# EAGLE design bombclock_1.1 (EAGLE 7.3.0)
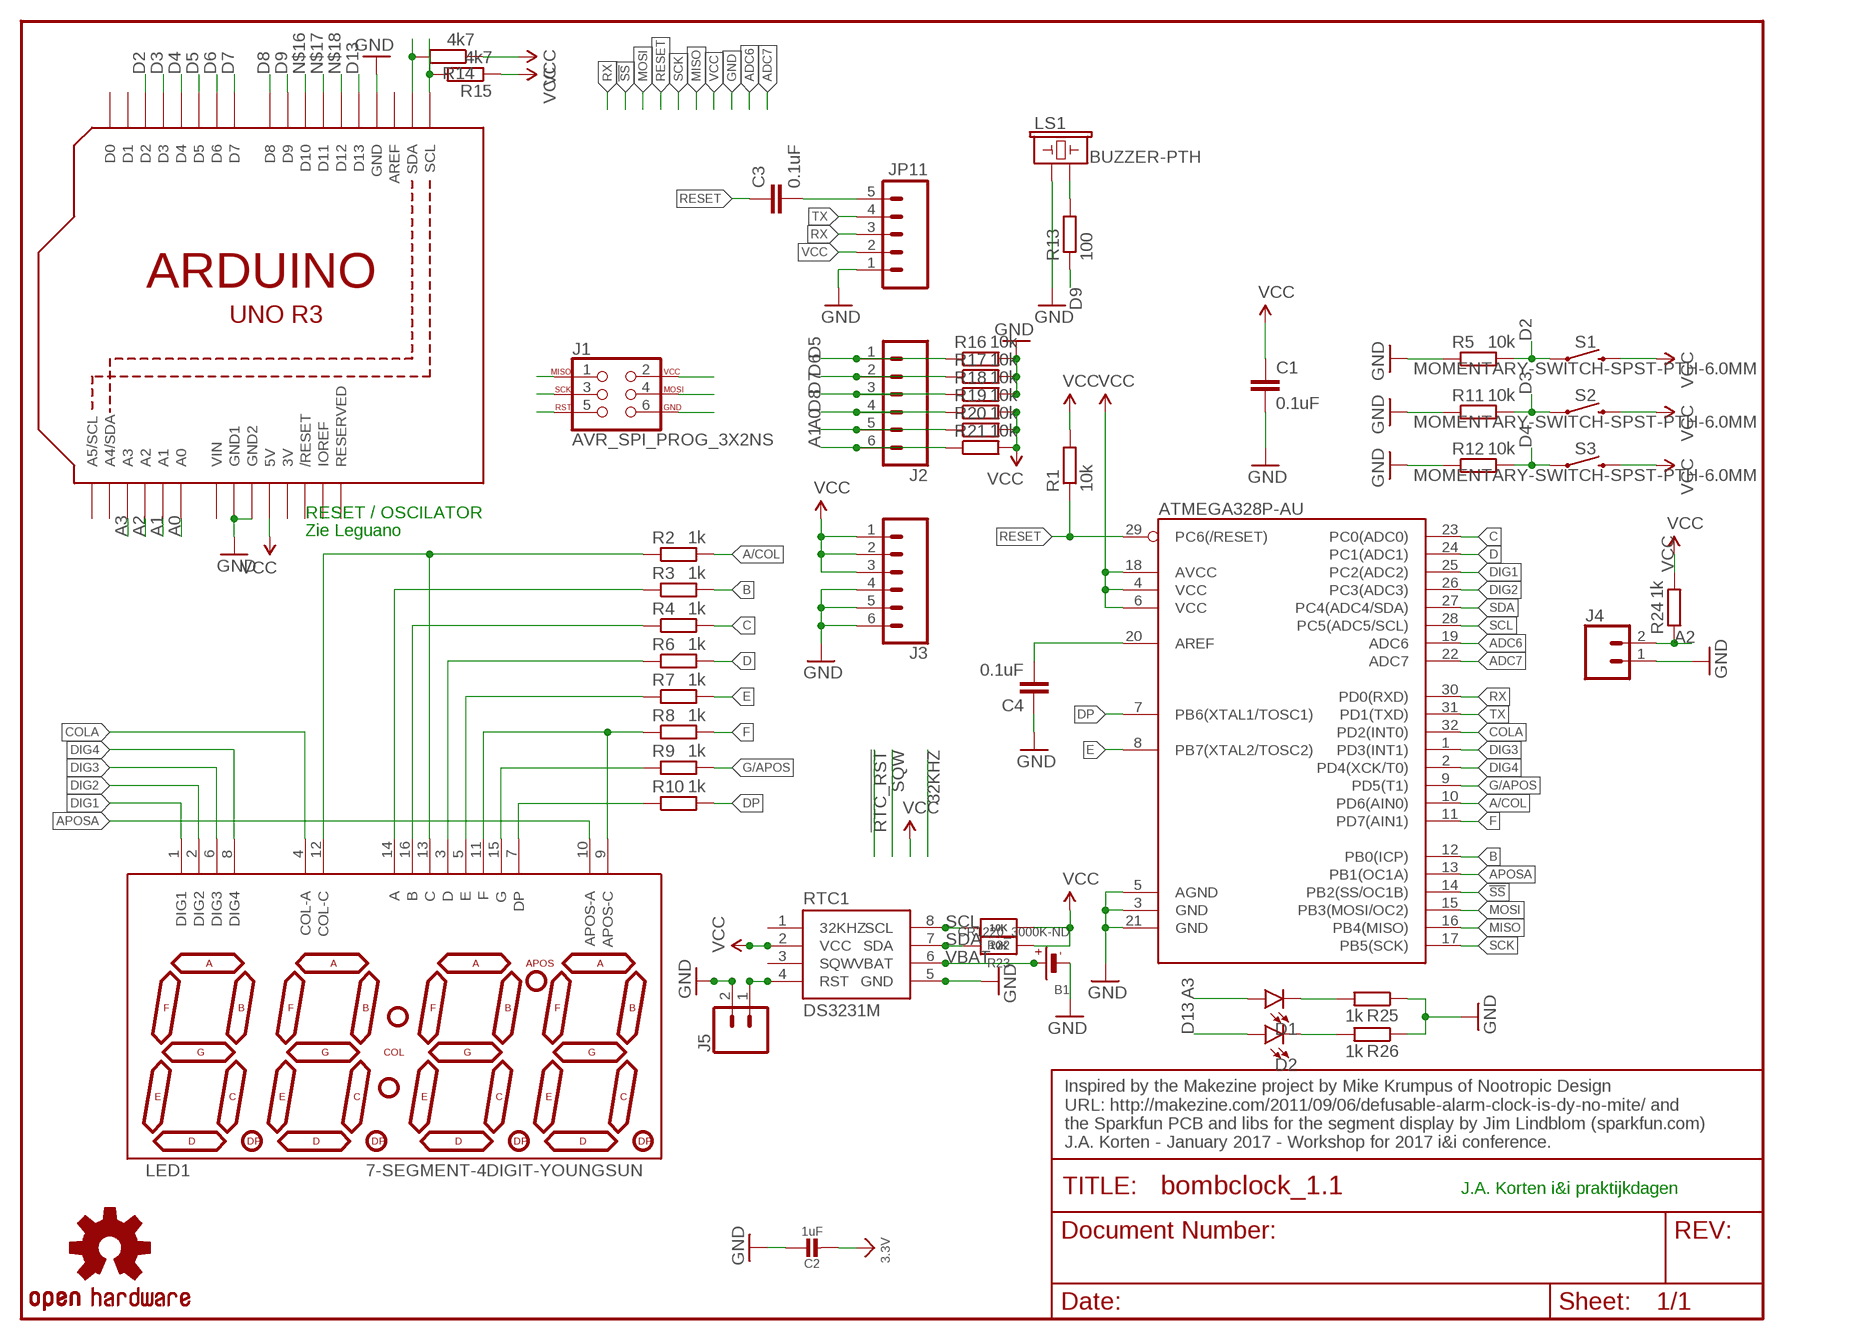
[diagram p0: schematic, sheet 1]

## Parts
ATMEGA328P-AU  ATMEGA328P-AU  ATMEGA168  [TQFP32-08]
B1  CR1220_3000K-ND  BATTERYCR1220_SMT  [CR1220]
C1  0.1uF  CAP0402-CAP  [0402-CAP]
C2  1uF  CAP_CERAMIC0805-NOOUTLINE  [0805-NO]
C3  0.1uF  CAP0402-CAP  [0402-CAP]
C4  0.1uF  CAP0402-CAP  [0402-CAP]
D1  LED5MM  [LED_5MM]
D2  LED5MM  [LED_5MM]
J1  AVR_SPI_PROG_3X2NS  [2X3-NS]
J2  CONN_06SILK_FEMALE_PTH  [1X06]
J3  CONN_06SILK_FEMALE_PTH  [1X06]
J4  CONN_02  [1X02]
J5  CONN_02  [1X02]
JP11  M05PTH-NS  [1X05_NO_SILK]
LED1  7-SEGMENT-4DIGIT-YOUNGSUN  [7-SEGMENT-4DIGIT-YOUNGSUN]
LS1  BUZZER-PTH  [BUZZER-12MM]
R1  10k  R-EU_R0603  [R0603]
R2  1k  R-EU_R0603  [R0603]
R3  1k  R-EU_R0603  [R0603]
R4  1k  R-EU_R0603  [R0603]
R5  10k  R-EU_R0603  [R0603]
R6  1k  R-EU_R0603  [R0603]
R7  1k  R-EU_R0603  [R0603]
R8  1k  R-EU_R0603  [R0603]
R9  1k  R-EU_R0603  [R0603]
R10  1k  R-EU_R0603  [R0603]
R11  10k  R-EU_R0603  [R0603]
R12  10k  R-EU_R0603  [R0603]
R13  100  R-EU_R0603  [R0603]
R14  4k7  R-EU_R0603  [R0603]
R15  4k7  R-EU_R0603  [R0603]
R16  10k  R-EU_R0603  [R0603]
R17  10k  R-EU_R0603  [R0603]
R18  10k  R-EU_R0603  [R0603]
R19  10k  R-EU_R0603  [R0603]
R20  10k  R-EU_R0603  [R0603]
R21  10k  R-EU_R0603  [R0603]
R22  10K  RESISTOR0805_NOOUTLINE  [0805-NO]
R23  10K  RESISTOR0805_NOOUTLINE  [0805-NO]
R24  1k  R-EU_R0603  [R0603]
R25  1k  R-EU_R0603  [R0603]
R26  1k  R-EU_R0603  [R0603]
RTC1  DS3231M  [SO08]
S1  MOMENTARY-SWITCH-SPST-PTH-6.0MM  [TACTILE_SWITCH_PTH_6.0MM]
S2  MOMENTARY-SWITCH-SPST-PTH-6.0MM  [TACTILE_SWITCH_PTH_6.0MM]
S3  MOMENTARY-SWITCH-SPST-PTH-6.0MM  [TACTILE_SWITCH_PTH_6.0MM]
U1  ARDUINOR3-DIMENSION  [ARDUINOR3]
U$4  OSHW-LOGOS  [OSHW-LOGO-S]

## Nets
3.3V: C2.2
!SS: ATMEGA328P-AU.14(PB2(SS/OC1B))
A0: J2.5 R20.1 U1.A0
A1: J2.6 R21.1 U1.A1
A2: J4.2 R24.1 U1.A2
A3: D1.A U1.A3
A/COL: ATMEGA328P-AU.10(PD6(AIN0)) R2.2
ADC6: ATMEGA328P-AU.19(ADC6)
ADC7: ATMEGA328P-AU.22(ADC7)
APOSA: ATMEGA328P-AU.13(PB1(OC1A)) LED1.10(APOS-A)
B: ATMEGA328P-AU.12(PB0(ICP)) R3.2
C: ATMEGA328P-AU.23(PC0(ADC0)) R4.2
COLA: ATMEGA328P-AU.32(PD2(INT0)) LED1.4(COL-A)
D: ATMEGA328P-AU.24(PC1(ADC1)) R6.2
D2: R5.2 S1.1 U1.D2
D3: R11.2 S2.1 U1.D3
D4: R12.2 S3.1 U1.D4
D5: J2.1 R16.1 U1.D5
D6: J2.2 R17.1 U1.D6
D7: J2.3 R18.1 U1.D7
D8: J2.4 R19.1 U1.D8
D9: R13.1 U1.D9
D13: D2.A U1.D13
DIG1: ATMEGA328P-AU.25(PC2(ADC2)) LED1.1(DIG1)
DIG2: ATMEGA328P-AU.26(PC3(ADC3)) LED1.2(DIG2)
DIG3: ATMEGA328P-AU.1(PD3(INT1)) LED1.6(DIG3)
DIG4: ATMEGA328P-AU.2(PD4(XCK/T0)) LED1.8(DIG4)
DP: ATMEGA328P-AU.7(PB6(XTAL1/TOSC1)) R10.2
E: ATMEGA328P-AU.8(PB7(XTAL2/TOSC2)) R7.2
F: ATMEGA328P-AU.11(PD7(AIN1)) R8.2
G/APOS: ATMEGA328P-AU.9(PD5(T1)) R9.2
GND: ATMEGA328P-AU.3(GND) ATMEGA328P-AU.5(AGND) ATMEGA328P-AU.21(GND) B1.- C1.2 C2.1 C4.1 J1.6 J3.4 J3.5 J3.6 J4.1 J5.2 JP11.1 LS1.+ R5.1 R11.1 R12.1 R16.2 R17.2 R18.2 R25.1 R26.1 RTC1.5(GND) U1.GND U1.GND1 U1.GND2
MISO: ATMEGA328P-AU.16(PB4(MISO)) J1.1
MOSI: ATMEGA328P-AU.15(PB3(MOSI/OC2)) J1.4
N$1: ATMEGA328P-AU.20(AREF) C4.2
N$2: LED1.7(DP) R10.1
N$3: LED1.15(G) R9.1
N$4: LED1.9(APOS-C) LED1.11(F) R8.1
N$5: LED1.5(E) R7.1
N$6: LED1.3(D) R6.1
N$8: LED1.16(B) R4.1
N$9: LED1.14(A) R3.1
N$10: LED1.12(COL-C) LED1.13(C) R2.1
N$12: D1.K(C) R25.2
N$13: C3.2 JP11.5
N$14: D2.K(C) R26.2
N$16: U1.D10
N$17: U1.D11
N$18: U1.D12
N$20: LS1.- R13.2
PP: J5.1 RTC1.4(RST)
RESET: ATMEGA328P-AU.29(PC6(/RESET)) C3.1 J1.5 R1.1
RX: ATMEGA328P-AU.30(PD0(RXD)) JP11.3
SCK: ATMEGA328P-AU.17(PB5(SCK)) J1.3
SCL: ATMEGA328P-AU.28(PC5(ADC5/SCL)) R15.2 R22.2 RTC1.8(SCL) U1.SCL
SDA: ATMEGA328P-AU.27(PC4(ADC4/SDA)) R14.2 R23.2 RTC1.7(SDA) U1.SDA
TX: ATMEGA328P-AU.31(PD1(TXD)) JP11.4
VBAT: B1.+$1(+) RTC1.6(VBAT)
VCC: ATMEGA328P-AU.4(VCC) ATMEGA328P-AU.6(VCC) ATMEGA328P-AU.18(AVCC) C1.1 J1.2 J3.1 J3.2 J3.3 JP11.2 R1.2 R14.1 R15.1 R19.2 R20.2 R21.2 R22.1 R23.1 R24.2 RTC1.2(VCC) S1.3 S2.3 S3.3 U1.5V
Unconnected: RTC1.1(32KHZ) RTC1.3(SQW) U1.A4(A4/SDA) U1.A5(A5/SCL) U1.AREF U1.D0 U1.D1 U1.IOREF U1.RESERVED U1.RESET(/RESET)

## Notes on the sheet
- RESET / OSCILATOR
- Zie Leguano
- Inspired by the Makezine project by Mike Krumpus of Nootropic Design 
  URL: http://makezine.com/2011/09/06/defusable-alarm-clock-is-dy-no-mite/ and 
  the Sparkfun PCB and libs for the segment display by Jim Lindblom (sparkfun.com)
  J.A. Korten - January 2017 - Workshop for 2017 i&i conference.
- J.A. Korten i&i praktijkdagen

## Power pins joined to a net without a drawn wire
3V: U1.3V
VIN: U1.VIN

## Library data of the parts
ATMEGA328P-AU = SparkFun:ATMEGA168
B1 = microbuilder:BATTERY: CR1220 SMT - Digikey: 3001K-ND
C1 = SparkFun:CAP: Capacitor
C2 = microbuilder:CAP_CERAMIC: Ceramic Capacitors
C3 C4 = SparkFun-Passives:CAP: Capacitor
D1 D2 = SparkFun-LED:LED: LED (Generic)
J1 = SparkFun-Connectors:AVR_SPI_PROG_3X2: AVR ISP 6 Pin This is the reduced ISP connector for AVR programming. Common on Arduino. This footprint will take up less PCB space and can be used with a 10-pin to 6-pin adapter such as SKU: BOB-08508 **Special note about "TEST_POINT" package. The stop mask is on the top side, so if you want your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
J2 J3 = SparkFun-Connectors:CONN_06: Multi connection point. Often used as Generic Header-pin footprint for 0.1 inch spaced/style header connections On any of the 0.1 inch spaced packages, you can populate with these: Break Away Headers - Straight (PRT-00116) Break Away Male Headers - Right Angle (PRT-00553) Female Headers (PRT-00115)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; PROD_ID: CONN-08437
J4 J5 = SparkFun-Connectors:CONN_02: Multi connection point. Often used as Generic Header-pin footprint for 0.1 inch spaced/style header connections
JP11 = SparkFun-Connectors:M05: Header 5 Standard 5-pin 0.1" header. Use with straight break away headers (SKU : PRT-00116), right angle break away headers (PRT-00553), swiss pins (PRT-00743), machine pins (PRT-00117), and female headers (PRT-00115). Molex polarized connector foot print use with SKU : PRT-08230 with associated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
LED1 = SparkFun:7-SEGMENT-4DIGIT-YOUNGSUN: This is a part for the 4-Digit 7-segment LEDs from Young Sun. Different from the Digikey LEDs, all 16 pins are used. The LONGPADS Variant is used for a test jig, but you may like it because there is more pad to solder to. If you are concerned about routing space, the standard works just fine though.
LS1 = SparkFun-Electromechanical:BUZZER: Buzzer; PROD_ID: COMP-08253; SF_SKU: COM-07950
R1-R21 R24-R26 = rcl:R-EU_: RESISTOR, European symbol
R22 R23 = microbuilder:RESISTOR: Resistors
RTC1 = SparkFun-Clocks:DS3231M: DS3231M Real Time Clock Accuracy +/-5ppm. Battery Backup. 2.3V to 5.5V. Datasheet SparkFun Products CryptoCape (DEV-12773) SparkFun CryptoShield (DEV-13183); PROD_ID: IC-11985
S1-S3 = SparkFun-Switches:MOMENTARY-SWITCH-SPST: Momentary Switch (Pushbutton) - SPST; PROD_ID: SWCH-08441; SF_SKU: COM-00097
U1 = adafruit:ARDUINOR3: This is a new object for the new Arduino R3 - with extra pins that you may want to use (such as IOref, and duplicated A4/A5
U$4 = SparkFun-Aesthetics:OSHW-LOGO: Open Source Hardware Logo This logo indicates the piece of hardware it is found on incorporates a OSHW license and/or adheres to the definition of open source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

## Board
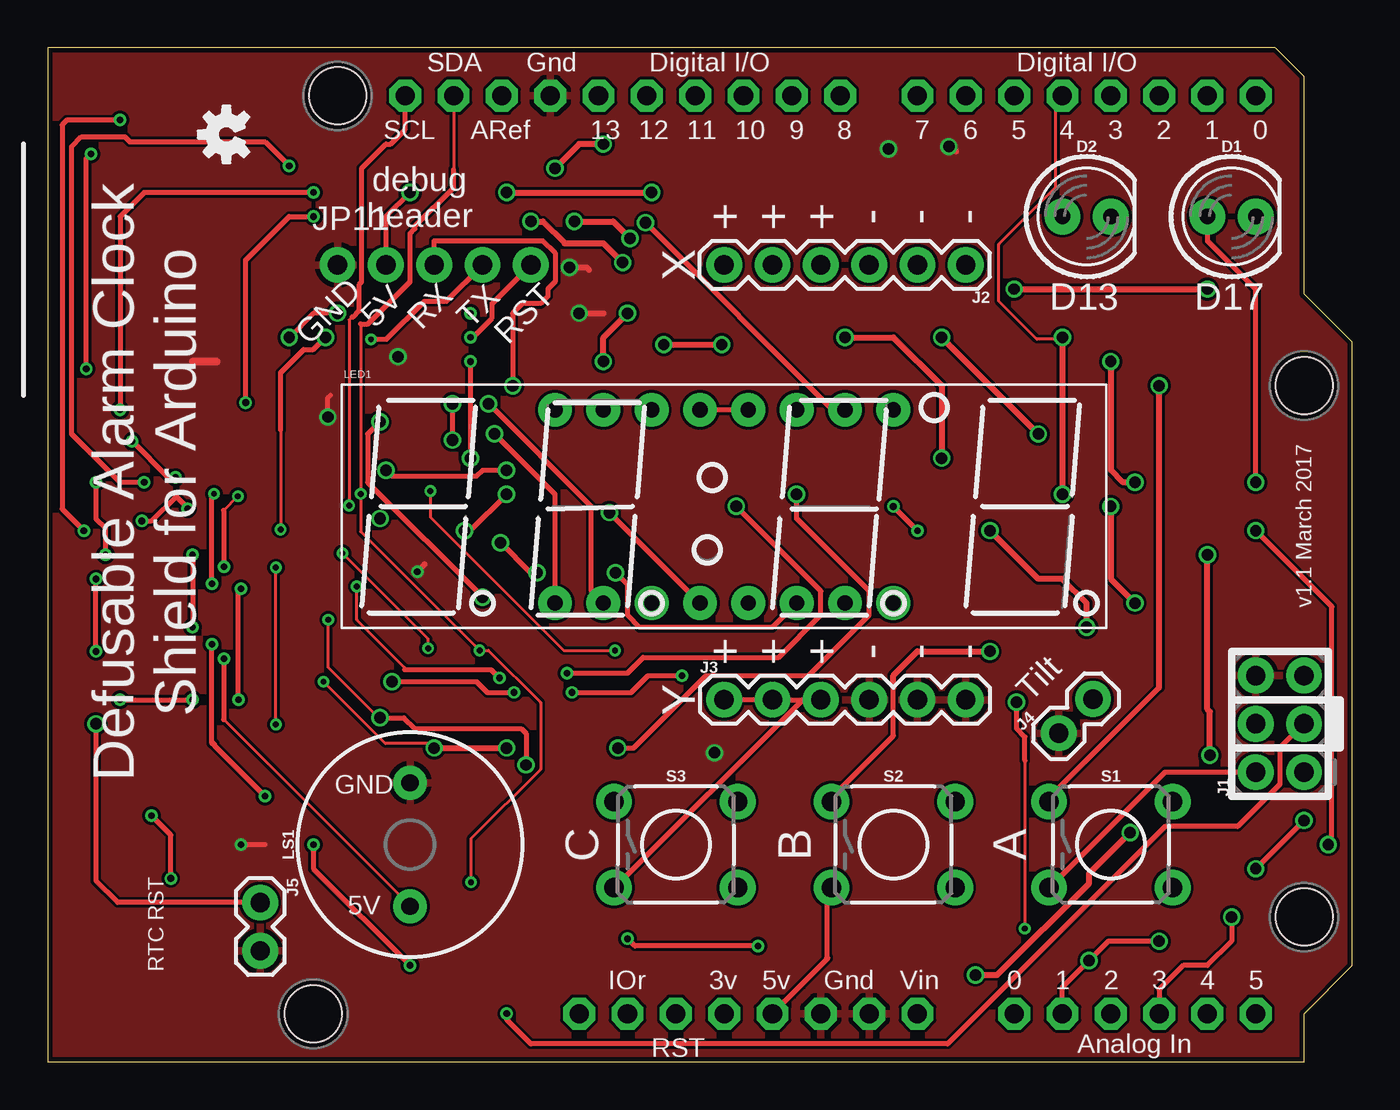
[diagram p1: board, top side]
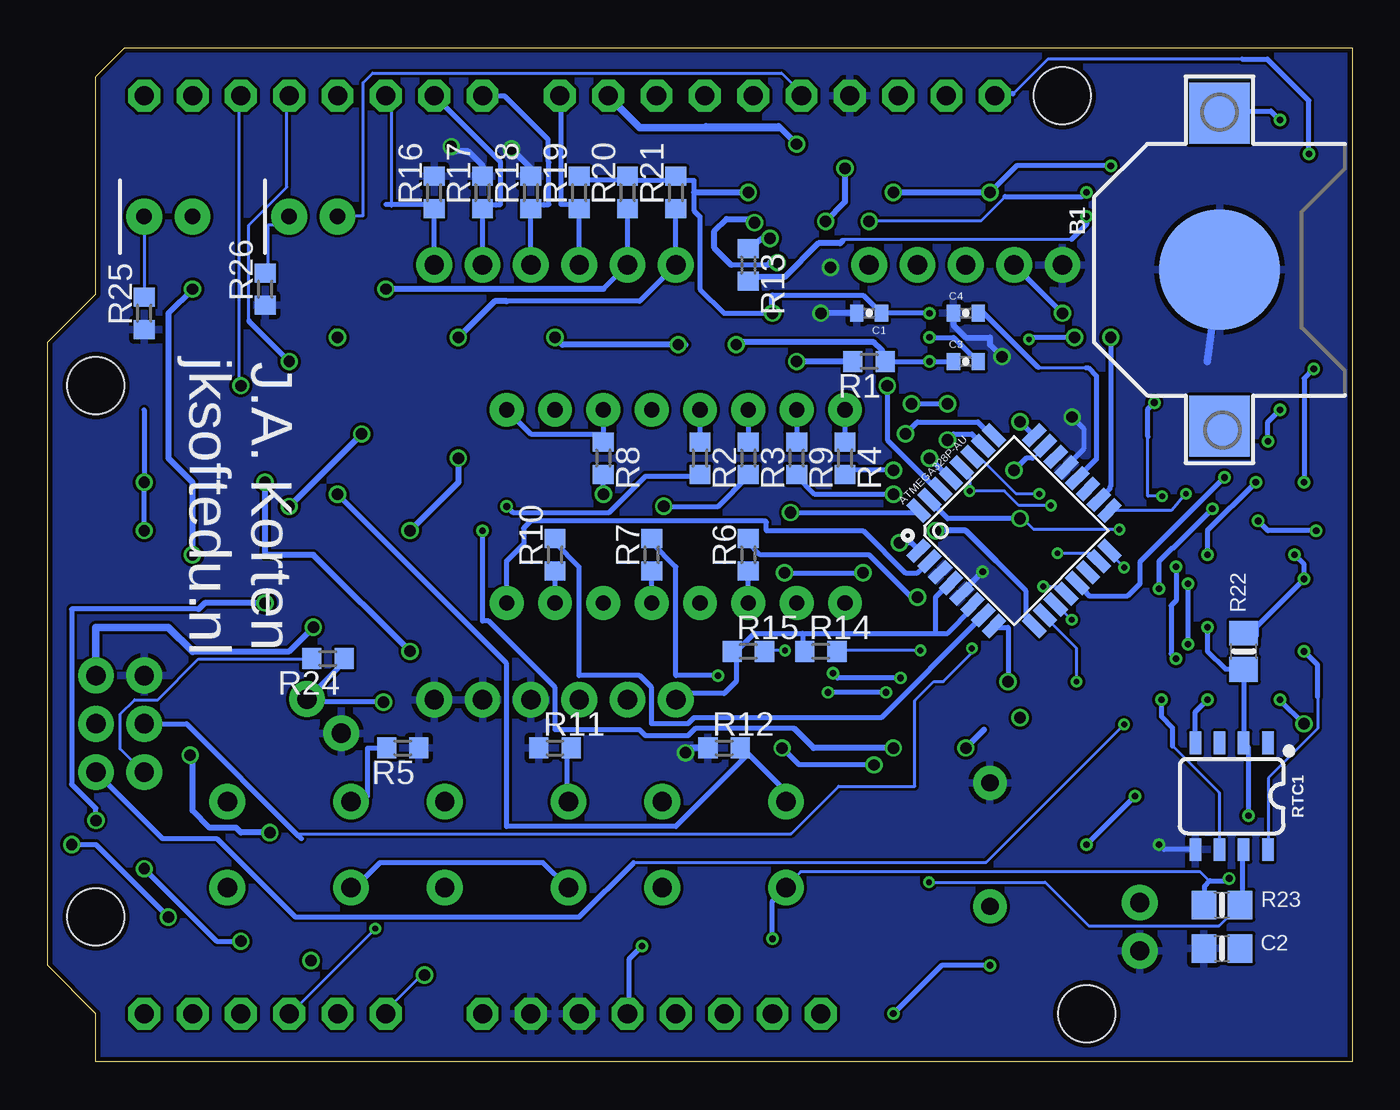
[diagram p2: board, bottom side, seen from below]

Size 68.58 x 53.34 mm. Coordinates in mm from the lower left corner, seen from the top.
Copper layers (1*16): Top 0.035mm / dielectric 1.5mm / Bottom 0.035mm
Design rules "ITEADstudioDRC": minimum track width 6mil, minimum drill 12mil, track to track 6mil, track to pad 6mil, pad to pad 6mil, via to via 6mil, smd to smd 0mil, copper to edge 10mil, drill to drill 10mil, minimum pad ring 10mil, minimum via ring 6mil, stop-mask expansion 2mil, vias tented up to drill 100mil, thermal gap 10mil
Holes 3 mm at 66.04,35.56 66.04,7.62 15.24,50.8 13.97,2.54

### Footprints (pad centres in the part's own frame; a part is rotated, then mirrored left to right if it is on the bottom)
TQFP32-08 = smd 1.27 x 0.559: 1 -4.293,2.8; 2 -4.293,2; 3 -4.293,1.2; 4 -4.293,0.4; 5 -4.293,-0.4; 6 -4.293,-1.2; 7 -4.293,-2; 8 -4.293,-2.8; 17 4.293,-2.8; 18 4.293,-2; 19 4.293,-1.2; 20 4.293,-0.4; 21 4.293,0.4; 22 4.293,1.2; 23 4.293,2; 24 4.293,2.8 | smd 0.559 x 1.27: 9 -2.8,-4.293; 10 -2,-4.293; 11 -1.2,-4.293; 12 -0.4,-4.293; 13 0.4,-4.293; 14 1.2,-4.293; 15 2,-4.293; 16 2.8,-4.293; 25 2.8,4.293; 26 2,4.293; 27 1.2,4.293; 28 0.4,4.293; 29 -0.4,4.293; 30 -1.2,4.293; 31 -2,4.293; 32 -2.8,4.293
CR1220 = smd 3.2 x 3.2: +$1 -8.225,0; +$2 8.225,0 | smd 6.35 x 6.35: - 0,0
0402-CAP = smd 0.7 x 0.9: 1 -0.65,0; 2 0.65,0
0805-NO = smd 1.3 x 1.5: 1 -0.95,0; 2 0.95,0
LED_5MM = drill 0.813 pad 1.88: A -1.27,0; K 1.27,0
2X3-NS = drill 1.016 pad 1.88: 1 -2.54,-1.27; 2 -2.54,1.27; 3 0,-1.27; 4 0,1.27; 5 2.54,-1.27; 6 2.54,1.27
1X06 = drill 1.016 pad 1.88: 1 0,0; 2 2.54,0; 3 5.08,0; 4 7.62,0; 5 10.16,0; 6 12.7,0
1X02 = drill 1.016 pad 1.88: 1 0,0; 2 2.54,0
1X05_NO_SILK = drill 1.016 pad 1.88: 1 0,0; 2 2.54,0; 3 5.08,0; 4 7.62,0; 5 10.16,0
7-SEGMENT-4DIGIT-YOUNGSUN = drill 0.8 pad 1.778: 1 -8.89,-5.08; 2 -6.35,-5.08; 3 -3.81,-5.08; 4 -1.27,-5.08; 5 1.27,-5.08; 6 3.81,-5.08; 7 6.35,-5.08; 8 8.89,-5.08; 9 8.89,5.08; 10 6.35,5.08; 11 3.81,5.08; 12 1.27,5.08; 13 -1.27,5.08; 14 -3.81,5.08; 15 -6.35,5.08; 16 -8.89,5.08
BUZZER-12MM = drill 0.9 pad 1.778: + 3.25,0; - -3.25,0
R0603 = smd 1 x 1.1: 1 -0.85,0; 2 0.85,0
SO08 = smd 0.6 x 1.2: 1 -1.905,-2.8; 2 -0.635,-2.8; 3 0.635,-2.8; 4 1.905,-2.8; 5 1.905,2.8; 6 0.635,2.8; 7 -0.635,2.8; 8 -1.905,2.8
TACTILE_SWITCH_PTH_6.0MM = drill 1.016 pad 1.88: 1 -3.251,2.261; 2 3.251,2.261; 3 -3.251,-2.261; 4 3.251,-2.261
ARDUINOR3 = drill 1 pad 1.676 octagon: 3V 35.56,2.54; 5V 38.1,2.54; A0 50.8,2.54; A1 53.34,2.54; A2 55.88,2.54; A3 58.42,2.54; A4 60.96,2.54; A5 63.5,2.54; AREF 23.876,50.8; D0 63.5,50.8; D1 60.96,50.8; D2 58.42,50.8; D3 55.88,50.8; D4 53.34,50.8; D5 50.8,50.8; D6 48.26,50.8; D7 45.72,50.8; D8 41.656,50.8; D9 39.116,50.8; D10 36.576,50.8; D11 34.036,50.8; D12 31.496,50.8; D13 28.956,50.8; GND 26.416,50.8; GND1 43.18,2.54; GND2 40.64,2.54; IOREF 30.48,2.54; RESERVED 27.94,2.54; RESET 33.02,2.54; SCL 18.796,50.8; SDA 21.336,50.8; VIN 45.72,2.54

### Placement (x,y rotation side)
ATMEGA328P-AU  17.78,27.94 45 bottom
B1  6.99,41.66 270 bottom
C1  25.4,39.37 180 bottom
C2  6.86,5.97 0 bottom
C3  20.32,36.83 0 bottom
C4  20.32,39.37 0 bottom
D1  62.23,44.45 0 top
D2  54.61,44.45 0 top
J1  64.77,17.78 90 top
J2  48.26,41.91 180 top
J3  35.56,19.05 0 top
J4  53.14,17.29 45 top
J5  11.18,8.38 270 top
JP11  15.24,41.91 0 top
LED1  35.56,29.21 0 top
LS1  19.05,11.43 90 top
R1  25.4,36.83 180 bottom
R2  34.29,31.75 270 bottom
R3  31.75,31.75 270 bottom
R4  26.67,31.75 270 bottom
R5  49.91,16.51 180 bottom
R6  31.75,26.67 90 bottom
R7  36.83,26.67 90 bottom
R8  39.37,31.75 270 bottom
R9  29.21,31.75 270 bottom
R10  41.91,26.67 90 bottom
R11  41.91,16.51 0 bottom
R12  33.02,16.51 0 bottom
R13  31.75,41.91 270 bottom
R14  27.94,21.59 0 bottom
R15  31.75,21.59 0 bottom
R16  48.26,45.72 90 bottom
R17  45.72,45.72 90 bottom
R18  43.18,45.72 90 bottom
R19  40.64,45.72 90 bottom
R20  38.1,45.72 90 bottom
R21  35.56,45.72 90 bottom
R22  5.71,21.59 90 bottom
R23  6.86,8.26 0 bottom
R24  53.85,21.21 180 bottom
R25  63.5,39.37 90 bottom
R26  57.15,40.64 90 bottom
RTC1  6.35,13.97 180 bottom
S1  55.88,11.43 0 top
S2  44.45,11.43 0 top
S3  33.02,11.43 0 top
U1  0,0 0 top
U$4  9.4,48.77 90 top

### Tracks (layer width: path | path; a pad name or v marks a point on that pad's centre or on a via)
A0  (via drill 0.6)
  Top 0.305: v50.8,40.64 v60.96,40.64 | v48.77,4.57 49.91,4.57 54.74,9.4 54.74,9.91 v56.9,12.06 | v61.09,16.13 61.09,18.41 60.96,18.54 v60.96,26.67
  Bottom 0.152: U1.A0 50.5,3 49,4.5 v48.77,4.57
  Bottom 0.254: R20.1 J2.5 39.37,40.64
  Bottom 0.305: 39.37,40.64 v50.8,40.64 | v60.96,40.64 62.23,39.37 62.23,31.75 60.96,30.48 v60.96,26.67 | v56.9,12.06 58.42,12.06 58.67,12.32 60.07,12.32 60.96,13.21 60.96,16 v61.09,16.13
A1  (via drill 0.6)
  Top 0.254: U1.A1 53.34,3.94 v54.74,5.33 55.75,6.35 v58.42,6.35 | v63.5,10.16 v66.04,12.7
  Top 0.305: v46.99,38.1 v52.07,33.02 | v55.88,29.21 55.88,25.4 v57.15,24.13
  Bottom 0.254: R21.1 J2.6 37.47,40.01 44.45,40.01 | 60.64,23.81 67.31,23.81 67.31,14.61 66.04,13.34 v66.04,12.7 | v63.5,10.16 59.69,6.35 v58.42,6.35
  Bottom 0.305: 44.45,40.01 45.09,40.01 v46.99,38.1 | v52.07,33.02 v55.88,29.21 | v57.15,24.13 60.33,24.13 60.64,23.81
A2  (via drill 0.3, 0.6)
  Top 0.152: 51.36,15.85 v51.36,7.01
  Top 0.254: 51.36,15.85 51.36,17.09 50.93,17.53 v50.93,18.92
  Bottom 0.152: 53.34,21.18 R24.1 | 54.56,19.05 J4.2 | v51.36,7.01 55.78,2.59 U1.A2
  Bottom 0.254: v50.93,18.92 54.78,18.92 J4.2 53.34,20.68 53.34,21.18
A3  (via drill 0.6)
  Top 0.254: v67.31,11.43 67.5,11.62 67.5,23.94 v63.5,27.94 | v62.23,7.62 62.23,6.35 60.96,5.08 59.69,5.08 58.42,3.81 U1.A3 | v63.5,30.48 63.5,40.64 60.96,43.18 D1.A
  Bottom 0.254: v67.31,11.43 66.04,11.43 v62.23,7.62 | v63.5,27.94 v63.5,30.48 63.5,34.29
A/COL  (via drill 0.3, 0.35, 0.6)
  Top 0.152: v14.5,20 17.75,16.75 20.25,16.75 v20.32,16.51
  Top 0.254: v44.45,29.21 v45.72,27.94
  Top 0.305: v20.32,16.51 v24.13,16.51
  Bottom 0.152: v14.5,20 14.5,21.75 16,23.25 ATMEGA328P-AU.10
  Bottom 0.254: v45.72,27.94 45.72,23.18 45.4,23.18 41.91,19.68 41.91,17.46 37.47,17.46 37.15,17.14 34.92,17.14 34.54,17.53 29.34,17.53 | R2.2 34.29,30.8 37.15,30.8 39.05,28.89 44.13,28.89 v44.45,29.21
  Bottom 0.305: 19.37,17.46 v20.32,16.51 | v24.13,16.51 28.32,16.51 29.34,17.53
APOSA  (via drill 0.35, 0.6, 0.61)
  Top 0.254: v31.43,44.13 41.27,34.29 LED1.10 | v13.97,45.72 5.08,45.72 3.81,44.45 v3.81,34.29 | v6.73,30.73 6.35,30.73 v4.45,32.64
  Top 0.305: v25.4,44.2 26.04,44.2 27.18,43.05 29.21,43.05 v30.23,42.04
  Bottom 0.152: 14,24.75 14.25,25 ATMEGA328P-AU.13 | 18.25,45.5 19.5,44.25 25.25,44.25 v25.4,44.2
  Bottom 0.254: 30.73,41.91 32.64,41.91 | 18.25,45.5 14.19,45.5 v13.97,45.72 | 14,24.75 14,24.67 13.84,24.51 11.81,24.51 11.18,25.15 11.18,26.29 v6.73,30.73 | v4.45,32.64 4.45,33.66 v3.81,34.29
  Bottom 0.305: 25.34,44.13 v25.4,44.2 | v30.23,42.04 30.61,42.04 30.73,41.91 | 32.64,41.91 33.53,42.8 33.53,43.69 32.89,44.32 31.62,44.32 v31.43,44.13
B  (via drill 0.3, 0.35, 0.61)
  Top 0.152: v16.25,25 16.25,23.25 18.75,20.75 18.75,20.64
  Top 0.254: v36.2,29.21 40.64,24.77 40.64,23.5 38.42,21.27 31.3,21.27 30.48,20.45 v27.3,20.45 | 18.75,20.64 23.3,20.64 v23.75,20.19
  Bottom 0.152: v16.25,25 15.5,25 15.25,24.75 ATMEGA328P-AU.12
  Bottom 0.254: v36.2,29.21 33.34,29.21 31.75,30.8 R3.2 | v23.75,20.19 27.05,20.19 v27.3,20.45
C  (via drill 0.61)
  Top 0.254: v24.13,31.11 22.86,31.11 22.54,30.8 18.1,30.8 v17.78,31.11
  Bottom 0.152: ATMEGA328P-AU.23 16.25,32.25 16.75,31.75 16.83,31.75
  Bottom 0.254: v24.13,31.11 26.67,31.11 R4.2 | v17.78,31.11 17.14,31.75 16.83,31.75
COLA  (via drill 0.61)
  Top 0.254: LED1.4 v29.53,28.89
  Bottom 0.254: v29.53,28.89 22.86,28.89 ATMEGA328P-AU.32
D  (via drill 0.61)
  Top 0.254: v22.86,24.45 16.83,30.48 16.83,33.02 v17.46,33.66
  Bottom 0.254: v22.86,24.45 23.18,24.45 25.4,26.67 31.11,26.67 31.75,27.3 R6.2 | v17.46,33.66 16.83,33.02 ATMEGA328P-AU.24
D2  (via drill 0.6)
  Top 0.254: 58.42,19.68 52.7,13.97 S1.1
  Top 0.305: 58.42,19.68 v58.42,35.56
  Bottom 0.152: U1.D2 58.5,50.5 58.5,36 v58.42,35.56
  Bottom 0.254: R5.2 51.75,16.51 51.75,13.97 52.39,13.97 S1.1
D3  (via drill 0.6)
  Top 0.254: 44.45,19.68 44.45,17.14 41.27,13.97 S2.1
  Top 0.305: 44.45,19.68 44.45,20.32 45.72,21.59 v49.53,21.59 | v57.15,30.48 56.52,30.48 55.88,31.11 v55.88,36.83
  Bottom 0.152: 58,39 58,44 56,46 56,50.5 U1.D3
  Bottom 0.254: R11.2 41.27,16.51 41.27,13.97 S2.1 | 58,39 58,38.95 v55.88,36.83
  Bottom 0.305: v49.53,21.59 54.61,26.67 57.15,26.67 v57.15,30.48
D4  (via drill 0.6, 0.61)
  Top 0.152: U1.D4 53,50.5 53,46 50,43 50,40 52,38 53,38 v53.34,38.1
  Top 0.305: v53.34,38.1 v53.34,29.84
  Bottom 0.152: 53.5,50.5 U1.D4 | 53.5,38.5 v53.34,38.1
  Bottom 0.254: 31.75,16.19 32.07,16.51 R12.2 | S3.1 29.53,13.97 31.75,16.19 | v53.34,29.84 44.45,20.95 44.45,12.38 35.56,12.38 31.75,16.19
D5
  Bottom 0.152: U1.D5 50.5,50.5 50.5,45.09 50.5,45
  Bottom 0.254: J2.1 R16.1 48.26,45.09 50.5,45.09 50.8,45.09
D6
  Bottom 0.152: 45,45 45,45.09
  Bottom 0.254: J2.2 R17.1 45.72,45.09 45,45.09 44.77,45.09 44.77,47.31 U1.D6
D7
  Bottom 0.152: 42.5,45 42.5,45.09
  Bottom 0.254: J2.3 R18.1 43.18,45.09 42.5,45.09 42.23,45.09 42.23,47.31 42.29,47.37 42.29,48.51 44.58,50.8 U1.D7
D8
  Bottom 0.152: U1.D8 41.5,50.5 41.59,50.5
  Bottom 0.254: J2.4 R19.1 40.64,45.09 41.59,45.09 41.59,50.5 41.59,50.8
D9  (via drill 0.6)
  Top 0.305: v29.21,48.26 27.94,48.26 v26.67,46.99 | v27.69,44.2 29.72,44.2 v30.61,43.31
  Bottom 0.152: U1.D9 39,50.5 37.5,49 30,49 29.98,49.02
  Bottom 0.254: 33.97,49.21 37.47,49.21 39.05,50.8
  Bottom 0.305: 33.97,49.21 30.16,49.21 29.98,49.02 v29.21,48.26 | v26.67,46.99 26.67,45.21 v27.69,44.2 | v30.61,43.31 31,43.31 R13.1
D13
  Bottom 0.152: U1.D13 29,51 30,52 51.5,52 52,51.5 52,44.5 53,44.5 D2.A
DIG1  (via drill 0.61)
  Top 0.254: v23.5,33.02 26.67,29.84 LED1.1
  Bottom 0.254: v23.5,33.02 22.86,33.66 19.68,33.66 19.05,33.02 ATMEGA328P-AU.25
DIG2  (via drill 0.61)
  Top 0.254: v21.27,34.61 v21.27,32.7 | v23.18,34.61 28.57,29.21 28.57,24.77 LED1.2
  Bottom 0.254: v21.27,32.7 20.95,33.02 20,33.02 19.68,32.7 ATMEGA328P-AU.26 | v23.18,34.61 v21.27,34.61
DIG3  (via drill 0.61)
  Top 0.254: v23.81,27.3 25.4,25.72 v25.72,25.72 | v29.84,25.72 30.48,25.08 30.48,23.5 31.11,22.86 38.1,22.86 LED1.6
  Bottom 0.254: v23.81,27.3 23.18,27.3 22.86,26.99 ATMEGA328P-AU.1 | v29.84,25.72 v25.72,25.72
DIG4
  Bottom 0.254: LED1.8 44.45,26.35 43.56,27.24 43.56,28.07 43.18,28.45 30.86,28.45 30.8,28.38 30.8,27.94 25.72,27.94 23.5,25.72 22.86,25.72 22.54,26.04 ATMEGA328P-AU.2
DP
  Bottom 0.254: R10.2 41.91,27.3 40.64,26.04 40.64,20.32 37.47,20.32 36.83,19.68 36.83,17.78 34.92,17.78 34.61,18.1 24.77,18.1 19.68,23.18 ATMEGA328P-AU.7
E  (via drill 0.35, 0.61)
  Top 0.254: v33.34,20.32 31.56,20.32 30.67,19.43 v27.56,19.43 | v18.1,20 22.54,20 23.11,19.43 v24.51,19.43
  Bottom 0.254: v33.34,20.32 35.56,20.32 35.56,26.04 36.83,27.3 R7.2 | v18.1,20 18.1,22.86 18.73,22.86 ATMEGA328P-AU.8 | v24.51,19.43 v27.56,19.43
F  (via drill 0.3, 0.6, 0.61)
  Top 0.152: v14.75,23.25 14.75,20.75 17.25,18.25 v17.46,18.1
  Top 0.254: v39.37,29.84 39.37,28.57 43.18,24.77 43.18,23.5 40.01,20.32 34.61,20.32 30.8,16.51 v29.97,16.51 | v17.46,18.1 18.73,18.1 19.3,17.53 24.89,17.53 25.15,17.27 v25.15,15.62
  Bottom 0.152: v14.75,23.25 15.5,24 ATMEGA328P-AU.11
  Bottom 0.254: v39.37,29.84 R8.2 | v25.15,15.62 29.08,15.62 v29.97,16.51
G/APOS  (via drill 0.61)
  Top 0.254: v24.13,29.84 22.23,27.94 v21.91,27.94
  Bottom 0.254: v24.13,29.84 28.26,29.84 29.21,30.8 R9.2 | 18.73,26.35 17.14,24.77 17.14,23.18 16.83,23.18 ATMEGA328P-AU.9
  Bottom 0.305: 18.73,26.35 20.32,27.94 v21.91,27.94
GND  (via drill 0.35, 0.6)
  Top 0.254: v14.73,33.91 14.73,34.92 14.86,35.05 | v10.16,11.43 11.43,11.43
  Top 0.305: v27.94,39.37 29.21,39.37 | v47.37,48.13 47.5,48.13 47.75,47.88 | v44.2,48.01 44.2,47.88 44.07,47.75 | v35.05,16.26 35.05,16 | v19.43,25.78 19.81,26.16 | v27.43,41.78 28.32,41.78 28.45,41.66
  Top 0.406: 7.62,36.83 8.89,36.83
  Bottom 0.254: ATMEGA328P-AU.21 15.03,31.33 14.1,32.26 14.1,33.27 v14.73,33.91 | RTC1.5 9.9,11.17 v10.16,11.43
  Bottom 0.305: C1.2 v27.94,39.37 | R17.2 45.72,47.12 46.48,47.88 47.12,47.88 v47.37,48.13 | R18.2 43.18,46.99 v44.2,48.01 | R12.1 34.8,16.51 v35.05,16.26 | ATMEGA328P-AU.5 20.53,24.68 v19.43,25.78 | C4.1 20.97,38.75 20.32,38.1 19.05,38.1 19.05,37.72 v18.41,37.08
  Bottom 0.406: B1.- 7.62,36.83
  pour Bottom: 0,53.34 68.58,53.34 68.58,0 0,0
  pour Top: 0,0 0,53.34 68.58,53.34 68.58,0
MISO  (via drill 0.3)
  Top 0.152: v12,17.75 v12,26
  Bottom 0.152: v12,26 12.75,26.75 ATMEGA328P-AU.16 | v12,17.75 19.25,10.5 37.75,10.5 37.78,10.48
  Bottom 0.254: 37.78,10.48 40.64,7.62 55.56,7.62 59.69,11.75 62.55,11.75 J1.1
MOSI  (via drill 0.3)
  Top 0.152: v15.5,26.75 20,22.25 v20,21.75
  Bottom 0.152: v15.5,26.75 13.75,26.75 13.5,26.5 ATMEGA328P-AU.15 | 55.5,12 29.5,12 27,14.5 23,14.5 23,19 22,20 21.5,20 20,21.5 v20,21.75
  Bottom 0.254: 55.24,11.75 55.5,12 61.28,17.78 J1.4
N$1
  Bottom 0.152: 14,36.5 16.5,36.5 16.51,36.51 | 14.25,30.75 ATMEGA328P-AU.20
  Bottom 0.254: 16.51,36.51 19.37,39.37 C4.2 | 14,36.5 13.89,36.5 13.46,36.07 13.46,31.69 ATMEGA328P-AU.20
N$2
  Bottom 0.254: LED1.7 R10.1
N$3
  Bottom 0.254: LED1.15 R9.1
N$4
  Bottom 0.254: LED1.11 39.37,33.02 | 39.37,33.02 R8.1 | 39.37,33.02 43.18,33.02 LED1.9
N$5
  Bottom 0.254: LED1.5 R7.1
N$6
  Bottom 0.254: LED1.3 R6.1
N$8
  Bottom 0.254: LED1.16 R4.1
N$9
  Bottom 0.254: LED1.14 R3.1
N$10
  Top 0.254: LED1.12 LED1.13
  Bottom 0.254: LED1.13 R2.1
N$12
  Bottom 0.152: D1.K R25.2 63.5,40
N$13  (via drill 0.35)
  Top 0.254: v22.23,38.1 22.35,38.1 23.37,39.12 23.37,39.88 JP11.5
  Bottom 0.254: v22.23,38.1 20.95,38.1 19.68,36.83 C3.2
N$14
  Bottom 0.152: R26.2 57,41.5 57,44 56,44 D2.K
N$20  (via drill 0.3, 0.35)
  Top 0.152: 9.25,29 v10,29.75 | 9.25,18 19,8.25 LS1.-
  Top 0.254: 19.05,8.26 LS1.- | v10.41,34.67 10.41,42.16 12.7,44.45 v13.97,44.45 | 9.25,29 9.25,26.06 v9.27,26.04 | v9.27,21.21 9.27,18.02 9.25,18
  Bottom 0.152: 14.77,43.25 26.75,43.25 26.8,43.18 | 10.75,32.88 10.75,29.75 v10,29.75
  Bottom 0.254: 31.75,41.27 R13.2 | 10.75,32.88 10.75,34.34 v10.41,34.67 | 14.77,43.25 13.97,44.05 v13.97,44.45 | v9.27,26.04 9.27,24.26 9.53,24 9.53,21.46 v9.27,21.21
  Bottom 0.305: 26.8,43.18 26.92,43.05 28.07,43.05 29.84,41.27 31.73,41.27 R13.2
PP  (via drill 0.35, 0.6)
  Top 0.254: v2.54,17.78 2.54,9.53 3.68,8.38 J5.1 | v3.81,19.05 v7.62,19.05
  Bottom 0.254: RTC1.4 8.26,18.41 v7.62,19.05 | v3.81,19.05 v2.54,17.78
RESET  (via drill 0.35, 0.6, 0.61)
  Top 0.254: v22.23,36.83 v22.23,31.75
  Top 0.305: v54.61,22.86 54.61,24.13 53.34,25.4 52.07,25.4 v49.53,27.94 | v32.38,37.72 v35.43,37.72 | v41.91,38.1 44.45,38.1 46.99,35.56 v46.99,31.75
  Bottom 0.254: R1.1 v22.23,36.83 C3.1 | v22.23,31.75 21.27,30.8 ATMEGA328P-AU.29
  Bottom 0.305: 60.96,21.59 55.88,21.59 v54.61,22.86 | R1.1 24.75,37.45 25.15,37.85 32.26,37.85 v32.38,37.72 | 35.05,37.72 v35.43,37.72 41.53,37.72 v41.91,38.1 | v46.99,31.75 46.99,30.48 v49.53,27.94
  Bottom 0.406: J1.5 66.04,22.86 62.23,22.86 60.96,21.59
RX  (via drill 0.61)
  Top 0.254: v24.45,35.56 24.45,39.37 24.96,39.88 25.91,39.88 26.29,40.26 26.29,40.64 26.67,41.02 26.67,42.55 26.04,43.18 20.32,43.18 JP11.3
  Bottom 0.254: v24.45,35.56 24.45,32.7 21.91,30.16 ATMEGA328P-AU.30
SCK  (via drill 0.3, 0.35)
  Top 0.254: J1.3 64.77,16.51 64.77,14.61 62.55,12.38 58.74,12.38 47.31,0.95 25.4,0.95 24.13,2.22 v24.13,2.54 | v11.43,13.97 8.75,16.65 8.75,16.75 8.64,16.75 v8.64,21.97 | v13.97,11.43 13.97,10.16 v19.05,5.08 | v8.64,25.15 8.64,29.77 v8.75,29.88
  Bottom 0.152: v8.75,29.88 9.5,29 ATMEGA328P-AU.17
  Bottom 0.254: v11.43,13.97 v13.97,11.43 | v19.05,5.08 21.59,5.08 v24.13,2.54 | v8.64,21.97 v8.64,25.15
SCL  (via drill 0.3, 0.35)
  Top 0.152: v29.82,21.64 27.13,21.64 20.12,28.65 v20.12,30.02 | v15.85,29.26 15.85,39.01 16,39.17
  Top 0.254: v2.54,21.59 v2.54,25.4 | v2.54,30.48 2.54,28.57 3.05,28.07 v3.05,26.67 | v2.03,36.45 2.03,47.5 v2.29,47.75 | 16,39.17 16.05,39.17 16.38,39.5 16.38,40.89 16.51,41.02 16.51,46.99 17.78,48.26 18.03,48.26 18.8,49.02 U1.SCL
  Bottom 0.152: v29.82,21.64 31.09,21.64 R15.2 | ATMEGA328P-AU.28 20.42,31.24 20.12,30.94 v20.12,30.02 18.29,30.02 17.53,29.26 v15.85,29.26 | 1.83,19.2 1.83,17.53 4.42,14.94 4.42,11.28 RTC1.8 | 17.83,50.9 16,52.73 5.79,52.73 | 18.75,50.9 U1.SCL | 5.64,22.4 5.03,22.4 R22.2 5.64,22.4
  Bottom 0.254: 1.83,19.2 1.83,20.88 v2.54,21.59 | v3.05,26.67 2.54,26.16 v2.54,25.4 5.03,22.91 5.03,22.4 | v2.54,30.48 2.54,35.94 v2.03,36.45 | v2.29,47.75 2.29,50.55 4.47,52.73 5.79,52.73 | 17.83,50.9 18.69,50.9 U1.SCL
SDA  (via drill 0.3)
  Top 0.152: 16.46,38.81 v16.46,29.87 16.46,27.89 v22.71,21.64 23.16,21.64 25.91,18.9 25.91,15.39 22.25,11.73 v22.25,9.45 | U1.SDA 21.34,46.94
  Top 0.254: 21.34,46.94 21.34,45.97 19.3,43.94 19.3,43.81 19.05,43.56 19.05,41.02 16.84,38.81 16.46,38.81
  Bottom 0.152: v22.71,21.64 27.28,21.64 R14.2 | v16.46,29.87 17.68,29.87 19.51,31.7 19.96,31.7 ATMEGA328P-AU.27 | v22.25,9.45 16.15,9.45 13.87,7.16 7.01,7.16 5.94,8.23 R23.2 5.79,8.38 | 5.79,11.12 RTC1.7
  Bottom 0.254: 5.79,11.12 5.79,8.37 R23.2
TX  (via drill 0.3, 0.6, 0.61)
  Top 0.152: 12.25,33.25 v12.25,28
  Top 0.254: 12.25,33.25 12.25,36.25 13.46,37.47 13.97,37.47 v14.61,38.1 | v17,38 17.81,38 19.81,40.01 20.95,40.01 JP11.4
  Bottom 0.152: v12.25,28 16.75,28 17.25,28.5 v17.46,28.57
  Bottom 0.254: v17.46,28.57 21.27,28.57 22.23,29.53 ATMEGA328P-AU.31 | v14.61,38.1 16.9,38.1 v17,38
VBAT  (via drill 0.35)
  Top 0.254: v10.03,19.05 10.03,24.77 v10.16,24.89 | v3.81,49.53 1.02,49.53 0.76,49.28 0.76,29.08 v1.91,27.94 | v4.95,28.45 5.46,28.45 6.76,29.74 7.37,29.13 v7.37,29.08
  Bottom 0.152: 7.5,50 B1.+$1 | 9.45,16.61 7.01,14.17 7.01,11.28 RTC1.6
  Bottom 0.254: 9.45,16.61 9.45,17.58 10.03,18.16 v10.03,19.05 | v10.16,24.89 10.16,26.34 9.5,27 9.45,27 v7.37,29.08 | 7.5,50 4.28,50 v3.81,49.53 | v1.91,27.94 4.45,27.94 v4.95,28.45
VCC  (via drill 0.35, 0.6)
  Top 0.152: 38.5,3 U1.5V | 41,5.5 40.96,5.5
  Top 0.254: 40.96,5.4 40.96,5.5 40.96,8.89 S2.3 | J1.2 58.74,15.24 52.7,9.21 S1.3 | J3.1 J3.2 39.69,19.05 | 39.69,19.05 J3.3 | 39.69,19.05 29.84,9.21 S3.3 | v15.24,39.37 13.97,39.37 v12.7,38.1 | v6.48,9.65 6.48,11.94 v5.46,12.95 | v5.08,30.48 3.81,30.48 1.27,33.02 1.27,48.13 1.78,48.64 4.06,48.64 4.32,48.39 11.43,48.39 v12.7,47.12 | 41,5.5 41,5.44 U1.5V | v37.34,6.1 30.86,6.1 v30.48,6.48 | v7.62,26.67 v7.62,22.86 | v19.05,45.72 17.78,44.45 JP11.2
  Top 0.305: v29.21,36.83 29.21,38.1 v30.48,39.37 | v24.13,45.72 v31.75,45.72
  Bottom 0.152: 38,3 U1.5V | 30,9 S3.3 29.5,9.5 29,10 8,10 7.5,9.5 7.49,9.53 | 13.25,29.75 ATMEGA328P-AU.18 | R24.2 54.56,21.18 60.66,21.18 62.79,19.05 64.01,19.05 64.77,18.29 64.77,16.46 63.55,15.24 J1.2 | 7.77,8.38 R23.1
  Bottom 0.254: 29.84,8.89 S3.3 30.48,8.46 v30.48,6.48 | S1.3 52.39,9.21 51.12,10.48 42.55,10.48 41.27,9.21 S2.3 | 26.04,36.83 R1.2 | 38.1,46.35 35.56,46.35 | 38.1,46.35 40.64,46.35 R19.2 | 38.1,46.35 R20.2 | 30.48,40.32 25.72,40.32 24.77,39.37 C1.1 v22.23,39.37 | 35.56,46.35 34.61,46.35 34.61,45.72 34.61,44.77 34.29,44.45 34.29,40.64 33.02,39.37 v30.48,39.37 | 35.56,46.35 R21.2 | 28.89,22.54 28.89,21.59 R14.1 | 28.89,22.54 31.43,22.54 32.38,21.59 | 28.89,22.54 21.91,22.54 | 21.91,22.54 21.27,22.54 20,23.81 ATMEGA328P-AU.6 | 21.91,22.54 21.91,24.45 21.27,25.08 ATMEGA328P-AU.4 | J3.1 35.24,19.37 33.02,19.37 32.38,20 32.38,21.59 | 32.38,21.59 R15.1 | v12.7,38.1 12.7,30.3 12.75,30.25 12.75,30.14 ATMEGA328P-AU.18 | 7.77,8.38 7.77,9.25 7.49,9.53 6.6,9.53 v6.48,9.65 | v5.46,12.95 5.46,16.52 RTC1.2 R22.1 6.67,20.64 7.62,21.59 v7.62,22.86 | v5.08,30.48 7.62,27.94 v7.62,26.67 | v12.7,47.12 17.65,47.12 v19.05,45.72 | 38,3 38,5.43 v37.34,6.1 | v15.24,39.37 JP11.2
  Bottom 0.305: 26.04,36.83 v29.21,36.83 | v30.48,39.37 30.48,40.32 | v19.05,45.72 v24.13,45.72 | v31.75,45.72 34.61,45.72

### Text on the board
_tsilk: debug / header | + | + | + | - | - | - | X | 5V | RX | TX | D13 | D17 | GND | RST | Defusable Alarm Clock / Shield for Arduino | v1.1 March 2017 | + | + | + | - | - | - | Tilt | Y | GND | C | B | A | 5V | RTC RST
_bsilk: J.A. Korten / jksoftedu.nl

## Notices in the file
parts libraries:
SparkFun-Electromechanical: Licensing: Creative Commons ShareAlike 4.0 International - https://creativecommons.org/licenses/by-sa/4.0
SparkFun-Connectors: Licensing: CC v3.0 Share-Alike You are welcome to use this library for commercial purposes.
